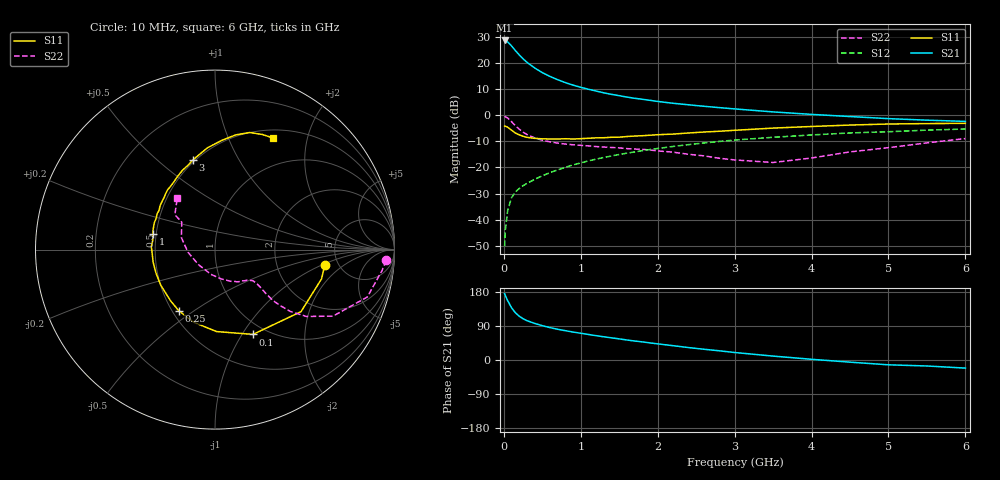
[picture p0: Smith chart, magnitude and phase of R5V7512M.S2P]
! SIEMENS Small Signal Semiconductors
! BFR183
! Si NPN RF Bipolar Junction Transistor in SOT23
! VCE = 0.75 V  IC = 12 mA
! Common Emitter S-Parameters:  May  1996
# GHz  S  MA  R  50
!  f  S11  S21  S12  S22
! GHz  MAG  ANG  MAG  ANG  MAG  ANG  MAG  ANG
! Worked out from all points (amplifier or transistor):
!   36 points, 10 MHz to 6 GHz, reference 50 ohm
!   highest |S21| = 28.7 dB at 10 MHz (marker M1)
!   |S21| within 3 dB of that: start of sweep to 125.2 MHz
!   unconditionally stable (mu >= 1): 576.4 MHz to 2.906 GHz
!   at 250 MHz: K = 0.71, MSG = 24.3 dB, |S12| = -27.0 dB
!   at 1.4 GHz: K = 1.09, MAG = 10.0 dB, |S12| = -15.6 dB
!   at 6 GHz: K = 0.96, MSG = 1.5 dB, |S12| = -5.3 dB
!   S11 on the Smith chart (normalised r, x): 10 MHz: 3.93, -1.07; 100 MHz: 0.87, -1.12; 250 MHz: 0.54, -0.44; 1 GHz: 0.48, +0.09; 3 GHz: 0.49, +0.66; 6 GHz: 0.60, +1.48
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0.01  0.6181 -7.8  27.19 175.2  0.0031 86.6  0.9543 -3.6
0.02  0.6155 -15.4  27.09 169.9  0.0063 82.9  0.9377 -7.2
0.05  0.5909 -35.8  25.45 156.4  0.015 75.6  0.8886 -17.3
0.1  0.5176 -65.9  21.35 138.1  0.0263 65.9  0.755 -29.4
0.15  0.4567 -88.9  17.37 124.6  0.0339 61.0  0.6307 -36.2
0.2  0.422 -106.1  14.39 115.7  0.0395 59.5  0.5429 -39.4
0.25  0.3961 -120.6  12.09 108.8  0.0448 58.8  0.4758 -40.7
0.3  0.3776 -131.0  10.39 103.8  0.0494 59.6  0.4283 -41.3
0.4  0.3615 -146.9  8.095 96.6  0.0591 61.1  0.3691 -40.7
0.5  0.3537 -158.6  6.568 90.6  0.0693 62.4  0.3325 -39.8
0.6  0.3517 -168.6  5.551 85.5  0.0795 63.3  0.309 -39.3
0.7  0.3504 -175.6  4.804 81.1  0.0899 63.5  0.2929 -39.2
0.8  0.3553 177.3  4.228 77.3  0.1009 63.4  0.2809 -39.3
1  0.3564 166.2  3.44 70.5  0.1223 63.2  0.2657 -40.2
1.1  0.3626 161.8  3.155 67.3  0.1334 62.6  0.2591 -41.6
1.6  0.3921 141.2  2.232 52.8  0.188 58.7  0.2296 -49.3
2.2  0.436 123.0  1.699 37.8  0.2527 52.0  0.1964 -64.0
3  0.5155 103.7  1.325 19.8  0.3351 41.4  0.1394 -99.5
3.5  0.5684 94.3  1.161 10.3  0.3787 34.4  0.1246 -137.8
4.5  0.6498 79.7  0.946 -5.7  0.4588 20.9  0.1989 160.3
5.5  0.6935 67.6  0.806 -15.8  0.5194 9.3  0.2962 139.0
6  0.7012 62.4  0.764 -21.4  0.5457 1.7  0.358 125.9
